| IBIS file stm32h523_533_lqfp100.ibs
[IBIS ver] 4.2
[File name] stm32h523_533_lqfp100.ibs
[File Rev] 0.2
[Date] 07-05-2024
[Source] Data Created at STMicroelectronics
[Notes]  File originated from ELDO simulations.
[Disclaimer]  This information is for modeling purpose only and is
   not guaranteed. The information is subject to change without
   notice.
[Copyright] Copyright 2024 STMicroelectronics Inc.
|   Component stm32h523_533_lqfp100
[Component] stm32h523_533_lqfp100
[Manufacturer] STMicroelectronics
[Package]
| variable   typ   min   max
R_pkg  0  NA  NA
L_pkg  0  NA  NA
C_pkg  0  NA  NA
[Pin]   signal_name   model_name
1  PE2  io8_ft_i3c_spi
2  PE3  io8_ft_i3c_spi
3  PE4  io8_ft_i3c_spi
4  PE5  io8_ft_i3c_spi
5  PE6  io8_ft_i3c_spi
6  VBAT  power
7  PC13  io8_ft_i3c_spi_v33
8  PC14-OSC32_IN  io_ft_tamp
9  PC15-OSC32_OUT  io_ft_tamp
10  VSS  gnd
11  VDD  power
12  PH0-OSC_IN  io8_ft_i3c_spi
13  PH1-OSC_OUT  io8_ft_i3c_spi
14  NRST  ioreset_ft_v33
15  PC0  io8_ft_spi
16  PC1  io8_ft_spi
17  PC2  io8_ft_spi
18  PC3  io8_ft_spi
19  VSSA  nc
20  VREFM  nc
21  VREFP  nc
22  VDDA  nc
23  PA0  io8_ft_spi
24  PA1  io8_ft_spi_tamp
25  PA2  io8_ft_spi
26  PA3  io8_ft_spi
27  VSS  gnd
28  VDD  power
29  PA4  io8_ft_spi
30  PA5  io8_ft_spi
31  PA6  io8_ft_spi
32  PA7  io8_ft_spi
33  PC4  io8_ft_spi
34  PC5  io8_ft_spi
35  PB0  io8_ft_spi
36  PB1  io8_ft_spi
37  PB2  io8_ft_i3c_spi
38  PE7  io8_ft_i3c_spi
39  PE8  io8_ft_i3c_spi
40  PE9  io8_ft_i3c_spi
41  PE10  io8_ft_i3c_spi
42  PE11  io8_ft_i3c_spi
43  PE12  io8_ft_i3c_spi
44  PE13  io8_ft_i3c_spi
45  PE14  io8_ft_i3c_spi
46  PE15  io8_ft_i3c_spi
47  PB10  io8_ft_i3c_spi
48  VCAP  nc
49  VSS  gnd
50  VDD  power
51  PB12  io8_ft_i3c_spi
52  PB13  nc
53  PB14  nc
54  PB15  io8_ft_spi
55  PD8  io8_ft_i3c_spi
56  PD9  io8_ft_i3c_spi
57  PD10  io8_ft_i3c_spi
58  PD11  io8_ft_i3c_spi
59  PD12  io8_ft_i3c_spi
60  PD13  io8_ft_i3c_spi
61  PD14  io8_ft_i3c_spi
62  PD15  io8_ft_i3c_spi
63  PC6  io8_ft_i3c_spi
64  PC7  io8_ft_i3c_spi
65  PC8  io8_ft_i3c_spi
66  PC9  io8_ft_i3c_spi
67  PA8  io8_ft_i3c_spi
68  PA9  io8_ft_i3c_spi
69  PA10  io8_ft_i3c_spi
70  PA11  io8usb_ft_i3c_spi_phy
71  PA12  io8usb_ft_i3c_spi_phy
72  PA13  io8_ft_i3c_spi
73  VDDUSB  power
74  VSS  gnd
75  VDD  power
76  PA14  io8_ft_i3c_spi
77  PA15  io8_ft_i3c_spi
78  PC10  io8_ft_i3c_spi
79  PC11  io8_ft_i3c_spi
80  PC12  io8_ft_i3c_spi
81  PD0  io8_ft_i3c_spi
82  PD1  io8_ft_i3c_spi
83  PD2  io8_ft_i3c_spi
84  PD3  io8_ft_i3c_spi
85  PD4  io8_ft_i3c_spi
86  PD5  io8_ft_i3c_spi
87  PD6  io8_ft_i3c_spi
88  PD7  io8_ft_i3c_spi
89  PB3  io8_ft_i3c_spi
90  PB4  io8_ft_i3c_spi
91  PB5  io8_ft_i3c_spi
92  PB6  io8_ft_i3c_spi
93  PB7  io8_ft_i3c_spi
94  BOOT0  vpphv
95  PB8  io8_ft_i3c_spi
96  PB9  io8_ft_i3c_spi
97  PE0  io8_ft_i3c_spi
98  VCAP  nc
99  VSS  gnd
100  VDD  power
[Package Model]   478-lqfp-14x14-100-240318
[Pin Mapping]   pulldown_ref   pullup_ref   | Comment
1  gndio  vddio
2  gndio  vddio
3  gndio  vddio
4  gndio  vddio
5  gndio  vddio
6  nc  vsw
7  gndio  vddio  | Depending on IO usage
| 7  gndio  vsw  | Depending on IO usage
8  gndio  vddio  | Depending on IO usage
| 8  gndio  vsw  | Depending on IO usage
9  gndio  vddio  | Depending on IO usage
| 9  gndio  vsw  | Depending on IO usage
10  gndio  nc
11  nc  vddio
12  gndio  vddio
13  gndio  vddio
14  gndio  vddio
15  gndio  vddio
16  gndio  vddio
17  gndio  vddio
18  gndio  vddio
19  nc  nc
20  nc  nc
21  nc  nc
22  nc  nc
23  gndio  vddio
24  gndio  vddio
25  gndio  vddio
26  gndio  vddio
27  gndio  nc
28  nc  vddio
29  gndio  vddio
30  gndio  vddio
31  gndio  vddio
32  gndio  vddio
33  gndio  vddio
34  gndio  vddio
35  gndio  vddio
36  gndio  vddio
37  gndio  vddio
38  gndio  vddio
39  gndio  vddio
40  gndio  vddio
41  gndio  vddio
42  gndio  vddio
43  gndio  vddio
44  gndio  vddio
45  gndio  vddio
46  gndio  vddio
47  gndio  vddio
48  nc  nc
49  gndio  nc
50  nc  vddio
51  gndio  vddio
52  nc  nc
53  nc  nc
54  gndio  vddio
55  gndio  vddio
56  gndio  vddio
57  gndio  vddio
58  gndio  vddio
59  gndio  vddio
60  gndio  vddio
61  gndio  vddio
62  gndio  vddio
63  gndio  vddio
64  gndio  vddio
65  gndio  vddio
66  gndio  vddio
67  gndio  vddio
68  gndio  vddio
69  gndio  vddio
70  gndio  vddusb  | Depending on IO usage
| 70  gndio  vddio  | Depending on IO usage
71  gndio  vddusb  | Depending on IO usage
| 71  gndio  vddio  | Depending on IO usage
72  gndio  vddio
73  nc  vddusb
74  gndio  nc
75  nc  vddio
76  gndio  vddio
77  gndio  vddio
78  gndio  vddio
79  gndio  vddio
80  gndio  vddio
81  gndio  vddio
82  gndio  vddio
83  gndio  vddio
84  gndio  vddio
85  gndio  vddio
86  gndio  vddio
87  gndio  vddio
88  gndio  vddio
89  gndio  vddio
90  gndio  vddio
91  gndio  vddio
92  gndio  vddio
93  gndio  vddio
94  gndio  vddio
95  gndio  vddio
96  gndio  vddio
97  gndio  vddio
98  nc  nc
99  gndio  nc
100  nc  vddio
|[Diff Pin]  inv_pin  vdiff  tdelay_typ  tdelay_min  tdelay_max
|71  70  NA  NA  NA  NA
[Model Selector] io8_ft_i3c_spi
io8_ft_spi_ls_1v2 "GPIO SPI - 5V tolerant - low speed - 1.2V range"
io8_ft_spi_ls_1v8 "GPIO SPI - 5V tolerant - low speed - 1.8V range"
io8_ft_spi_ls_3v3 "GPIO SPI - 5V tolerant - low speed - 3.3V range"
io8_ft_spi_ms_1v2 "GPIO SPI - 5V tolerant - med speed - 1.2V range"
io8_ft_spi_ms_1v8 "GPIO SPI - 5V tolerant - med speed - 1.8V range"
io8_ft_spi_ms_3v3 "GPIO SPI - 5V tolerant - med speed - 3.3V range"
io8_ft_spi_fs_1v2 "GPIO SPI - 5V tolerant - fast speed - 1.2V range"
io8_ft_spi_fs_1v8 "GPIO SPI - 5V tolerant - fast speed - 1.8V range"
io8_ft_spi_fs_3v3 "GPIO SPI - 5V tolerant - fast speed - 3.3V range"
io8_ft_spi_hs_1v2 "GPIO SPI - 5V tolerant - high speed - 1.2V range"
io8_ft_spi_hs_1v8 "GPIO SPI - 5V tolerant - high speed - 1.8V range"
io8_ft_spi_hs_3v3 "GPIO SPI - 5V tolerant - high speed - 3.3V range"
io8_ft_hslv_spi_ls_1v2 "GPIO SPI low volt opt - 5V tolerant - low speed - 1.2V range"
io8_ft_hslv_spi_ls_1v8 "GPIO SPI low volt opt - 5V tolerant - low speed - 1.8V range"
io8_ft_hslv_spi_ls_2v5 "GPIO SPI low volt opt - 5V tolerant - low speed - 2.5V range"
io8_ft_hslv_spi_ms_1v2 "GPIO SPI low volt opt - 5V tolerant - med speed - 1.2V range"
io8_ft_hslv_spi_ms_1v8 "GPIO SPI low volt opt - 5V tolerant - med speed - 1.8V range"
io8_ft_hslv_spi_ms_2v5 "GPIO SPI low volt opt - 5V tolerant - med speed - 2.5V range"
io8_ft_hslv_spi_fs_1v2 "GPIO SPI low volt opt - 5V tolerant - fast speed - 1.2V range"
io8_ft_hslv_spi_fs_1v8 "GPIO SPI low volt opt - 5V tolerant - fast speed - 1.8V range"
io8_ft_hslv_spi_fs_2v5 "GPIO SPI low volt opt - 5V tolerant - fast speed - 2.5V range"
io8_ft_hslv_spi_hs_1v2 "GPIO SPI low volt opt - 5V tolerant - high speed - 1.2V range"
io8_ft_hslv_spi_hs_1v8 "GPIO SPI low volt opt - 5V tolerant - high speed - 1.8V range"
io8_ft_hslv_spi_hs_2v5 "GPIO SPI low volt opt - 5V tolerant - high speed - 2.5V range"
io8_ft_i3c_spi_ls_1v2 "GPIO SPI with I3C open-drain - 5V tolerant - low speed - 1.2V range"
io8_ft_i3c_spi_ls_1v8 "GPIO SPI with I3C open-drain - 5V tolerant - low speed - 1.8V range"
io8_ft_i3c_spi_ls_3v3 "GPIO SPI with I3C open-drain - 5V tolerant - low speed - 3.3V range"
io8_ft_i3c_spi_ms_1v2 "GPIO SPI with I3C open-drain - 5V tolerant - med speed - 1.2V range"
io8_ft_i3c_spi_ms_1v8 "GPIO SPI with I3C open-drain - 5V tolerant - med speed - 1.8V range"
io8_ft_i3c_spi_ms_3v3 "GPIO SPI with I3C open-drain - 5V tolerant - med speed - 3.3V range"
io8_ft_i3c_spi_fs_1v2 "GPIO SPI with I3C open-drain - 5V tolerant - fast speed - 1.2V range"
io8_ft_i3c_spi_fs_1v8 "GPIO SPI with I3C open-drain - 5V tolerant - fast speed - 1.8V range"
io8_ft_i3c_spi_fs_3v3 "GPIO SPI with I3C open-drain - 5V tolerant - fast speed - 3.3V range"
io8_ft_i3c_spi_hs_1v2 "GPIO SPI with I3C open-drain - 5V tolerant - high speed - 1.2V range"
io8_ft_i3c_spi_hs_1v8 "GPIO SPI with I3C open-drain - 5V tolerant - high speed - 1.8V range"
io8_ft_i3c_spi_hs_3v3 "GPIO SPI with I3C open-drain - 5V tolerant - high speed - 3.3V range"
io8_ft_hslv_i3c_spi_ls_1v2 "GPIO SPI low volt opt with I3C open-drain - 5V tolerant - low speed - 1.2V range"
io8_ft_hslv_i3c_spi_ls_1v8 "GPIO SPI low volt opt with I3C open-drain - 5V tolerant - low speed - 1.8V range"
io8_ft_hslv_i3c_spi_ls_2v5 "GPIO SPI low volt opt with I3C open-drain - 5V tolerant - low speed - 2.5V range"
io8_ft_hslv_i3c_spi_ms_1v2 "GPIO SPI low volt opt with I3C open-drain - 5V tolerant - med speed - 1.2V range"
io8_ft_hslv_i3c_spi_ms_1v8 "GPIO SPI low volt opt with I3C open-drain - 5V tolerant - med speed - 1.8V range"
io8_ft_hslv_i3c_spi_ms_2v5 "GPIO SPI low volt opt with I3C open-drain - 5V tolerant - med speed - 2.5V range"
io8_ft_hslv_i3c_spi_fs_1v2 "GPIO SPI low volt opt with I3C open-drain - 5V tolerant - fast speed - 1.2V range"
io8_ft_hslv_i3c_spi_fs_1v8 "GPIO SPI low volt opt with I3C open-drain - 5V tolerant - fast speed - 1.8V range"
io8_ft_hslv_i3c_spi_fs_2v5 "GPIO SPI low volt opt with I3C open-drain - 5V tolerant - fast speed - 2.5V range"
io8_ft_hslv_i3c_spi_hs_1v2 "GPIO SPI low volt opt with I3C open-drain - 5V tolerant - high speed - 1.2V range"
io8_ft_hslv_i3c_spi_hs_1v8 "GPIO SPI low volt opt with I3C open-drain - 5V tolerant - high speed - 1.8V range"
io8_ft_hslv_i3c_spi_hs_2v5 "GPIO SPI low volt opt with I3C open-drain - 5V tolerant - high speed - 2.5V range"
io8_ft_i3c_fmp_spi_3v3 "GPIO SPI with I3C fm+ open-drain - 5V tolerant - 3.3V range"
io8_ft_i3c_fmp_spi_1v8 "GPIO SPI with I3C fm+ open-drain - 5V tolerant - 1.8V range"
io8_ft_i3c_fmp_spi_1v2 "GPIO SPI with I3C fm+ open-drain - 5V tolerant - 1.2V range"
[Model Selector] io8_ft_i3c_spi_v33
io8_ft_spi_v33_ls_1v2 ""GPIO SPI V33 - 5V tolerant - low speed - 1.2V range"
io8_ft_spi_v33_ls_1v8 ""GPIO SPI V33 - 5V tolerant - low speed - 1.8V range"
io8_ft_spi_v33_ls_3v3 ""GPIO SPI V33 - 5V tolerant - low speed - 3.3V range"
io8_ft_spi_v33_ms_1v2 ""GPIO SPI V33 - 5V tolerant - med speed - 1.2V range"
io8_ft_spi_v33_ms_1v8 ""GPIO SPI V33 - 5V tolerant - med speed - 1.8V range"
io8_ft_spi_v33_ms_3v3 ""GPIO SPI V33 - 5V tolerant - med speed - 3.3V range"
io8_ft_spi_v33_fs_1v2 ""GPIO SPI V33 - 5V tolerant - fast speed - 1.2V range
io8_ft_spi_v33_fs_1v8 ""GPIO SPI V33 - 5V tolerant - fast speed - 1.8V range
io8_ft_spi_v33_fs_3v3 ""GPIO SPI V33 - 5V tolerant - fast speed - 3.3V range
io8_ft_spi_v33_hs_1v2 ""GPIO SPI V33 - 5V tolerant - high speed - 1.2V range
io8_ft_spi_v33_hs_1v8 ""GPIO SPI V33 - 5V tolerant - high speed - 1.8V range
io8_ft_spi_v33_hs_3v3 ""GPIO SPI V33 - 5V tolerant - high speed - 3.3V range
io8_ft_hslv_spi_v33_ls_1v2 "GPIO SPI V33 low volt opt - 5V tolerant - low speed - 1.2V range""
io8_ft_hslv_spi_v33_ls_1v8 "GPIO SPI V33 low volt opt - 5V tolerant - low speed - 1.8V range""
io8_ft_hslv_spi_v33_ls_2v5 "GPIO SPI V33 low volt opt - 5V tolerant - low speed - 2.5V range""
io8_ft_hslv_spi_v33_ms_1v2 "GPIO SPI V33 low volt opt - 5V tolerant - med speed - 1.2V range""
io8_ft_hslv_spi_v33_ms_1v8 "GPIO SPI V33 low volt opt - 5V tolerant - med speed - 1.8V range""
io8_ft_hslv_spi_v33_ms_2v5 "GPIO SPI V33 low volt opt - 5V tolerant - med speed - 2.5V range""
io8_ft_hslv_spi_v33_fs_1v2 "GPIO SPI V33 low volt opt - 5V tolerant - fast speed - 1.2V range"
io8_ft_hslv_spi_v33_fs_1v8 "GPIO SPI V33 low volt opt - 5V tolerant - fast speed - 1.8V range"
io8_ft_hslv_spi_v33_fs_2v5 "GPIO SPI V33 low volt opt - 5V tolerant - fast speed - 2.5V range"
io8_ft_hslv_spi_v33_hs_1v2 "GPIO SPI V33 low volt opt - 5V tolerant - high speed - 1.2V range"
io8_ft_hslv_spi_v33_hs_1v8 "GPIO SPI V33 low volt opt - 5V tolerant - high speed - 1.8V range"
io8_ft_hslv_spi_v33_hs_2v5 "GPIO SPI V33 low volt opt - 5V tolerant - high speed - 2.5V range"
io8_ft_i3c_spi_v33_ls_1v2 "GPIO SPI V33 with I3C open-drain - 5V tolerant - low speed - 1.2V range"
io8_ft_i3c_spi_v33_ls_1v8 "GPIO SPI V33 with I3C open-drain - 5V tolerant - low speed - 1.8V range"
io8_ft_i3c_spi_v33_ls_3v3 "GPIO SPI V33 with I3C open-drain - 5V tolerant - low speed - 3.3V range"
io8_ft_i3c_spi_v33_ms_1v2 "GPIO SPI V33 with I3C open-drain - 5V tolerant - med speed - 1.2V range"
io8_ft_i3c_spi_v33_ms_1v8 "GPIO SPI V33 with I3C open-drain - 5V tolerant - med speed - 1.8V range"
io8_ft_i3c_spi_v33_ms_3v3 "GPIO SPI V33 with I3C open-drain - 5V tolerant - med speed - 3.3V range"
io8_ft_i3c_spi_v33_fs_1v2 "GPIO SPI V33 with I3C open-drain - 5V tolerant - fast speed - 1.2V range"
io8_ft_i3c_spi_v33_fs_1v8 "GPIO SPI V33 with I3C open-drain - 5V tolerant - fast speed - 1.8V range"
io8_ft_i3c_spi_v33_fs_3v3 "GPIO SPI V33 with I3C open-drain - 5V tolerant - fast speed - 3.3V range"
io8_ft_i3c_spi_v33_hs_1v2 "GPIO SPI V33 with I3C open-drain - 5V tolerant - high speed - 1.2V range"
io8_ft_i3c_spi_v33_hs_1v8 "GPIO SPI V33 with I3C open-drain - 5V tolerant - high speed - 1.8V range"
io8_ft_i3c_spi_v33_hs_3v3 "GPIO SPI V33 with I3C open-drain - 5V tolerant - high speed - 3.3V range"
io8_ft_hslv_i3c_spi_v33_ls_1v2 "GPIO SPI V33 low volt opt with I3C open-drain - 5V tolerant - low speed - 1.2V range"
io8_ft_hslv_i3c_spi_v33_ls_1v8 "GPIO SPI V33 low volt opt with I3C open-drain - 5V tolerant - low speed - 1.8V range"
io8_ft_hslv_i3c_spi_v33_ls_2v5 "GPIO SPI V33 low volt opt with I3C open-drain - 5V tolerant - low speed - 2.5V range"
io8_ft_hslv_i3c_spi_v33_ms_1v2 "GPIO SPI V33 low volt opt with I3C open-drain - 5V tolerant - med speed - 1.2V range"
io8_ft_hslv_i3c_spi_v33_ms_1v8 "GPIO SPI V33 low volt opt with I3C open-drain - 5V tolerant - med speed - 1.8V range"
io8_ft_hslv_i3c_spi_v33_ms_2v5 "GPIO SPI V33 low volt opt with I3C open-drain - 5V tolerant - med speed - 2.5V range"
io8_ft_hslv_i3c_spi_v33_fs_1v2 "GPIO SPI V33 low volt opt with I3C open-drain - 5V tolerant - fast speed - 1.2V range"
io8_ft_hslv_i3c_spi_v33_fs_1v8 "GPIO SPI V33 low volt opt with I3C open-drain - 5V tolerant - fast speed - 1.8V range"
io8_ft_hslv_i3c_spi_v33_fs_2v5 "GPIO SPI V33 low volt opt with I3C open-drain - 5V tolerant - fast speed - 2.5V range"
io8_ft_hslv_i3c_spi_v33_hs_1v2 "GPIO SPI V33 low volt opt with I3C open-drain - 5V tolerant - high speed - 1.2V range"
io8_ft_hslv_i3c_spi_v33_hs_1v8 "GPIO SPI V33 low volt opt with I3C open-drain - 5V tolerant - high speed - 1.8V range"
io8_ft_hslv_i3c_spi_v33_hs_2v5 "GPIO SPI V33 low volt opt with I3C open-drain - 5V tolerant - high speed - 2.5V range"
io8_ft_i3c_fmp_spi_v33_3v3 "GPIO SPI V33 with I3C fm+ open-drain - 5V tolerant - 3.3V range"
io8_ft_i3c_fmp_spi_v33_1v8 "GPIO SPI V33 with I3C fm+ open-drain - 5V tolerant - 1.8V range"
io8_ft_i3c_fmp_spi_v33_1v2 "GPIO SPI V33 with I3C fm+ open-drain - 5V tolerant - 1.2V range"
[Model Selector] io8_ft_spi
io8_ft_spi_ls_1v2 "GPIO SPI - 5V tolerant - low speed - 1.2V range"
io8_ft_spi_ls_1v8 "GPIO SPI - 5V tolerant - low speed - 1.8V range"
io8_ft_spi_ls_3v3 "GPIO SPI - 5V tolerant - low speed - 3.3V range"
io8_ft_spi_ms_1v2 "GPIO SPI- 5V tolerant - med speed - 1.2V range"
io8_ft_spi_ms_1v8 "GPIO SPI- 5V tolerant - med speed - 1.8V range"
io8_ft_spi_ms_3v3 "GPIO SPI- 5V tolerant - med speed - 3.3V range"
io8_ft_spi_fs_1v2 "GPIO SPI- 5V tolerant - fast speed - 1.2V range"
io8_ft_spi_fs_1v8 "GPIO SPI- 5V tolerant - fast speed - 1.8V range"
io8_ft_spi_fs_3v3 "GPIO SPI- 5V tolerant - fast speed - 3.3V range"
io8_ft_spi_hs_1v2 "GPIO SPI- 5V tolerant - high speed - 1.2V range"
io8_ft_spi_hs_1v8 "GPIO SPI- 5V tolerant - high speed - 1.8V range"
io8_ft_spi_hs_3v3 "GPIO SPI- 5V tolerant - high speed - 3.3V range"
io8_ft_hslv_spi_ls_1v2 "GPIO SPI low volt opt - 5V tolerant - low speed - 1.2V range"
io8_ft_hslv_spi_ls_1v8 "GPIO SPI low volt opt - 5V tolerant - low speed - 1.8V range"
io8_ft_hslv_spi_ls_2v5 "GPIO SPI low volt opt - 5V tolerant - low speed - 2.5V range"
io8_ft_hslv_spi_ms_1v2 "GPIO SPI low volt opt - 5V tolerant - med speed - 1.2V range"
io8_ft_hslv_spi_ms_1v8 "GPIO SPI low volt opt - 5V tolerant - med speed - 1.8V range"
io8_ft_hslv_spi_ms_2v5 "GPIO SPI low volt opt - 5V tolerant - med speed - 2.5V range"
io8_ft_hslv_spi_fs_1v2 "GPIO SPI low volt opt - 5V tolerant - fast speed - 1.2V range"
io8_ft_hslv_spi_fs_1v8 "GPIO SPI low volt opt - 5V tolerant - fast speed - 1.8V range"
io8_ft_hslv_spi_fs_2v5 "GPIO SPI low volt opt - 5V tolerant - fast speed - 2.5V range"
io8_ft_hslv_spi_hs_1v2 "GPIO SPI low volt opt - 5V tolerant - high speed - 1.2V range"
io8_ft_hslv_spi_hs_1v8 "GPIO SPI low volt opt - 5V tolerant - high speed - 1.8V range"
io8_ft_hslv_spi_hs_2v5 "GPIO SPI low volt opt - 5V tolerant - high speed - 2.5V range"
[Model Selector] io8_ft_spi_tamp
io8_ft_spi_ls_1v2 "GPIO SPI - 5V tolerant - low speed - 1.2V range"
io8_ft_spi_ls_1v8 "GPIO SPI - 5V tolerant - low speed - 1.8V range"
io8_ft_spi_ls_3v3 "GPIO SPI- 5V tolerant - low speed - 3.3V range"
io8_ft_spi_ms_1v2 "GPIO SPI - 5V tolerant - med speed - 1.2V range"
io8_ft_spi_ms_1v8 "GPIO SPI - 5V tolerant - med speed - 1.8V range"
io8_ft_spi_ms_3v3 "GPIO SPI - 5V tolerant - med speed - 3.3V range"
io8_ft_spi_fs_1v2 "GPIO SPI - 5V tolerant - fast speed - 1.2V range"
io8_ft_spi_fs_1v8 "GPIO SPI - 5V tolerant - fast speed - 1.8V range"
io8_ft_spi_fs_3v3 "GPIO SPI - 5V tolerant - fast speed - 3.3V range"
io8_ft_spi_hs_1v2 "GPIO SPI - 5V tolerant - high speed - 1.2V range"
io8_ft_spi_hs_1v8 "GPIO SPI - 5V tolerant - high speed - 1.8V range"
io8_ft_spi_hs_3v3 "GPIO SPI - 5V tolerant - high speed - 3.3V range"
io8_ft_hslv_spi_ls_1v2 "GPIO SPI low volt opt - 5V tolerant - low speed - 1.2V range"
io8_ft_hslv_spi_ls_1v8 "GPIO SPI low volt opt - 5V tolerant - low speed - 1.8V range"
io8_ft_hslv_spi_ls_2v5 "GPIO SPI low volt opt - 5V tolerant - low speed - 2.5V range"
io8_ft_hslv_spi_ms_1v2 "GPIO SPI low volt opt - 5V tolerant - med speed - 1.2V range"
io8_ft_hslv_spi_ms_1v8 "GPIO SPI low volt opt - 5V tolerant - med speed - 1.8V range"
io8_ft_hslv_spi_ms_2v5 "GPIO SPI low volt opt - 5V tolerant - med speed - 2.5V range"
io8_ft_hslv_spi_fs_1v2 "GPIO SPI low volt opt - 5V tolerant - fast speed - 1.2V range"
io8_ft_hslv_spi_fs_1v8 "GPIO SPI low volt opt - 5V tolerant - fast speed - 1.8V range"
io8_ft_hslv_spi_fs_2v5 "GPIO SPI low volt opt - 5V tolerant - fast speed - 2.5V range"
io8_ft_hslv_spi_hs_1v2 "GPIO SPI low volt opt - 5V tolerant - high speed - 1.2V range"
io8_ft_hslv_spi_hs_1v8 "GPIO SPI low volt opt - 5V tolerant - high speed - 1.8V range"
io8_ft_hslv_spi_hs_2v5 "GPIO SPI low volt opt - 5V tolerant - high speed - 2.5V range
io8_ft_tamp_v33_1v2 "IO tamper - 5V tolerant - 1.2V range"
io8_ft_tamp_v33_1v8 "IO tamper - 5V tolerant - 1.8V range"
io8_ft_tamp_v33_3v3 "IO tamper - 5V tolerant - 3.3V range"
[Model Selector] io8usb_ft_i3c_spi_phy
io8_ft_spi_ls_1v2 "GPIO SPI - 5V tolerant - low speed - 1.2V range"
io8_ft_spi_ls_1v8 "GPIO SPI - 5V tolerant - low speed - 1.8V range"
io8_ft_spi_ls_3v3 "GPIO SPI - 5V tolerant - low speed - 3.3V range"
io8_ft_spi_ms_1v2 "GPIO SPI - 5V tolerant - med speed - 1.2V range"
io8_ft_spi_ms_1v8 "GPIO SPI - 5V tolerant - med speed - 1.8V range"
io8_ft_spi_ms_3v3 "GPIO SPI - 5V tolerant - med speed - 3.3V range"
io8_ft_spi_fs_1v2 "GPIO SPI - 5V tolerant - fast speed - 1.2V range"
io8_ft_spi_fs_1v8 "GPIO SPI - 5V tolerant - fast speed - 1.8V range"
io8_ft_spi_fs_3v3 "GPIO SPI - 5V tolerant - fast speed - 3.3V range"
io8_ft_spi_hs_1v2 "GPIO SPI - 5V tolerant - high speed - 1.2V range"
io8_ft_spi_hs_1v8 "GPIO SPI - 5V tolerant - high speed - 1.8V range"
io8_ft_spi_hs_3v3 "GPIO SPI - 5V tolerant - high speed - 3.3V range"
io8_ft_hslv_spi_ls_1v2 "GPIO SPI low volt opt - 5V tolerant - low speed - 1.2V range"
io8_ft_hslv_spi_ls_1v8 "GPIO SPI low volt opt - 5V tolerant - low speed - 1.8V range"
io8_ft_hslv_spi_ls_2v5 "GPIO SPI low volt opt - 5V tolerant - low speed - 2.5V range"
io8_ft_hslv_spi_ms_1v2 "GPIO SPI low volt opt - 5V tolerant - med speed - 1.2V range"
io8_ft_hslv_spi_ms_1v8 "GPIO SPI low volt opt - 5V tolerant - med speed - 1.8V range"
io8_ft_hslv_spi_ms_2v5 "GPIO SPI low volt opt - 5V tolerant - med speed - 2.5V range"
io8_ft_hslv_spi_fs_1v2 "GPIO SPI low volt opt - 5V tolerant - fast speed - 1.2V range"
io8_ft_hslv_spi_fs_1v8 "GPIO SPI low volt opt - 5V tolerant - fast speed - 1.8V range"
io8_ft_hslv_spi_fs_2v5 "GPIO SPI low volt opt - 5V tolerant - fast speed - 2.5V range"
io8_ft_hslv_spi_hs_1v2 "GPIO SPI low volt opt - 5V tolerant - high speed - 1.2V range"
io8_ft_hslv_spi_hs_1v8 "GPIO SPI low volt opt - 5V tolerant - high speed - 1.8V range"
io8_ft_hslv_spi_hs_2v5 "GPIO SPI low volt opt - 5V tolerant - high speed - 2.5V range"
io8_ft_i3c_spi_ls_1v2 "GPIO SPI  with I3C open-drain - 5V tolerant - low speed - 1.2V range"
io8_ft_i3c_spi_ls_1v8 "GPIO SPI  with I3C open-drain - 5V tolerant - low speed - 1.8V range"
io8_ft_i3c_spi_ls_3v3 "GPIO SPI  with I3C open-drain - 5V tolerant - low speed - 3.3V range"
io8_ft_i3c_spi_ms_1v2 "GPIO SPI  with I3C open-drain - 5V tolerant - med speed - 1.2V range"
io8_ft_i3c_spi_ms_1v8 "GPIO SPI  with I3C open-drain - 5V tolerant - med speed - 1.8V range"
io8_ft_i3c_spi_ms_3v3 "GPIO SPI  with I3C open-drain - 5V tolerant - med speed - 3.3V range"
io8_ft_i3c_spi_fs_1v2 "GPIO SPI  with I3C open-drain - 5V tolerant - fast speed - 1.2V range"
io8_ft_i3c_spi_fs_1v8 "GPIO SPI  with I3C open-drain - 5V tolerant - fast speed - 1.8V range"
io8_ft_i3c_spi_fs_3v3 "GPIO SPI  with I3C open-drain - 5V tolerant - fast speed - 3.3V range"
io8_ft_i3c_spi_hs_1v2 "GPIO SPI  with I3C open-drain - 5V tolerant - high speed - 1.2V range"
io8_ft_i3c_spi_hs_1v8 "GPIO SPI  with I3C open-drain - 5V tolerant - high speed - 1.8V range"
io8_ft_i3c_spi_hs_3v3 "GPIO SPI  with I3C open-drain - 5V tolerant - high speed - 3.3V range"
io8_ft_hslv_i3c_spi_ls_1v2 "GPIO SPI  low volt opt with I3C open-drain - 5V tolerant - low speed - 1.2V range"
io8_ft_hslv_i3c_spi_ls_1v8 "GPIO SPI  low volt opt with I3C open-drain - 5V tolerant - low speed - 1.8V range"
io8_ft_hslv_i3c_spi_ls_2v5 "GPIO SPI  low volt opt with I3C open-drain - 5V tolerant - low speed - 2.5V range"
io8_ft_hslv_i3c_spi_ms_1v2 "GPIO SPI  low volt opt with I3C open-drain - 5V tolerant - med speed - 1.2V range"
io8_ft_hslv_i3c_spi_ms_1v8 "GPIO SPI  low volt opt with I3C open-drain - 5V tolerant - med speed - 1.8V range"
io8_ft_hslv_i3c_spi_ms_2v5 "GPIO SPI  low volt opt with I3C open-drain - 5V tolerant - med speed - 2.5V range"
io8_ft_hslv_i3c_spi_fs_1v2 "GPIO SPI  low volt opt with I3C open-drain - 5V tolerant - fast speed - 1.2V range"
io8_ft_hslv_i3c_spi_fs_1v8 "GPIO SPI  low volt opt with I3C open-drain - 5V tolerant - fast speed - 1.8V range"
io8_ft_hslv_i3c_spi_fs_2v5 "GPIO SPI  low volt opt with I3C open-drain - 5V tolerant - fast speed - 2.5V range"
io8_ft_hslv_i3c_spi_hs_1v2 "GPIO SPI  low volt opt with I3C open-drain - 5V tolerant - high speed - 1.2V range"
io8_ft_hslv_i3c_spi_hs_1v8 "GPIO SPI  low volt opt with I3C open-drain - 5V tolerant - high speed - 1.8V range"
io8_ft_hslv_i3c_spi_hs_2v5 "GPIO SPI  low volt opt with I3C open-drain - 5V tolerant - high speed - 2.5V range"
io8_ft_i3c_fmp_spi_3v3 "GPIO SPI  with I3C fm+ open-drain - 5V tolerant - 3.3V range"
io8_ft_i3c_fmp_spi_1v8 "GPIO SPI  with I3C fm+ open-drain - 5V tolerant - 1.8V range"
io8_ft_i3c_fmp_spi_1v2 "GPIO SPI  with I3C fm+ open-drain - 5V tolerant - 1.2V range"
io8usb_ft_phy_ls_2v5 "USB PHY - 5V tolerant - low speed - 2.5V range"
io8usb_ft_phy_ls_3v3 "USB PHY - 5V tolerant - low speed - 3.3V range
io8usb_ft_phy_fs_2v5 "USB PHY - 5V tolerant - fast speed - 2.5V range"
io8usb_ft_phy_fs_3v3 "USB PHY - 5V tolerant - fast speed - 3.3V range"
[Model Selector] io_ft_tamp
io_ft_tamp_3v3 "IO tamper - 5V tolerant - 3.3V range"
io_ft_tamp_1v8 "IO tamper - 5V tolerant - 1.8V range"
io_ft_tamp_1v2 "IO tamper - 5V tolerant - 1.2V range"
[Model Selector] ioreset_ft_v33
ioreset_ft_v33_1v2 "Reset PAD. 5V tolerant. 1.2V range"
ioreset_ft_v33_1v8 "Reset PAD. 5V tolerant. 1.8V range"
ioreset_ft_v33_3v3 "Reset PAD. 5V tolerant. 3.3V range"
[Model Selector] vpphv
vpphv_1v2 "Flash Test cell v33 = 1.2 V range"
vpphv_1v8 "Flash Test cell v33 = 1.8 V range"
vpphv_3v3 "Flash Test cell v33 = 3.3 V range"
[Define Package Model]  478-lqfp-14x14-100-240318
[Manufacturer]  Unknown
[OEM]  Unknown
[Description]  None
[Number Of Pins]  96
[Pin Numbers]
| Pin Num   Terminal Name
14 | NRST
23 | PA0
24 | PA1
25 | PA2
26 | PA3
29 | PA4
30 | PA5
31 | PA6
32 | PA7
67 | PA8
68 | PA9
69 | PA10
70 | PA11
71 | PA12
72 | PA13
76 | PA14
77 | PA15
35 | PB0
36 | PB1
37 | PB2
89 | PB3
90 | PB4
91 | PB5
92 | PB6
93 | PB7
95 | PB8
96 | PB9
47 | PB10
51 | PB12
52 | PB13
53 | PB14
54 | PB15
15 | PC0
16 | PC1
17 | PC2
18 | PC3
33 | PC4
34 | PC5
63 | PC6
64 | PC7
65 | PC8
66 | PC9
78 | PC10
79 | PC11
80 | PC12
7 | PC13
8 | PC14-OSC32_IN
9 | PC15-OSC32_OUT
81 | PD0
82 | PD1
83 | PD2
84 | PD3
85 | PD4
86 | PD5
87 | PD6
88 | PD7
55 | PD8
56 | PD9
57 | PD10
58 | PD11
59 | PD12
60 | PD13
61 | PD14
62 | PD15
97 | PE0
1 | PE2
2 | PE3
3 | PE4
4 | PE5
5 | PE6
38 | PE7
39 | PE8
40 | PE9
41 | PE10
42 | PE11
43 | PE12
44 | PE13
45 | PE14
46 | PE15
12 | PH0-OSC_IN
13 | PH1-OSC_OUT
6 | VBAT
48 | VCAP
98 | VCAP
50 | VDD
75 | VDD
11 | VDD
28 | VDD
100 | VDD
73 | VDDUSB
22 | VDDA
94 | BOOT0
20 | VREFM
21 | VREFP
10 | VSS
19 | VSSA
|[Merged Pins]  10
|27  |  VSS
|49  |  VSS
|74  |  VSS
|99  |  VSS
[Model Data]
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[End Model Data]
[End Package Model]
|End [Component]
| Models and submodels in the file (118): io8_ft_hslv_i3c_spi_fs_1v2 (I/O_open_drain), io8_ft_hslv_i3c_spi_fs_1v8 (I/O_open_drain), io8_ft_hslv_i3c_spi_fs_2v5 (I/O_open_drain), io8_ft_hslv_i3c_spi_hs_1v2 (I/O_open_drain), io8_ft_hslv_i3c_spi_hs_1v8 (I/O_open_drain), io8_ft_hslv_i3c_spi_hs_2v5 (I/O_open_drain), io8_ft_hslv_i3c_spi_ls_1v2 (I/O_open_drain), io8_ft_hslv_i3c_spi_ls_1v8 (I/O_open_drain), io8_ft_hslv_i3c_spi_ls_2v5 (I/O_open_drain), io8_ft_hslv_i3c_spi_ms_1v2 (I/O_open_drain), io8_ft_hslv_i3c_spi_ms_1v8 (I/O_open_drain), io8_ft_hslv_i3c_spi_ms_2v5 (I/O_open_drain), io8_ft_hslv_i3c_spi_v33_fs_1v2 (I/O_open_drain), io8_ft_hslv_i3c_spi_v33_fs_1v8 (I/O_open_drain), io8_ft_hslv_i3c_spi_v33_fs_2v5 (I/O_open_drain), io8_ft_hslv_i3c_spi_v33_hs_1v2 (I/O_open_drain), io8_ft_hslv_i3c_spi_v33_hs_1v8 (I/O_open_drain), io8_ft_hslv_i3c_spi_v33_hs_2v5 (I/O_open_drain), io8_ft_hslv_i3c_spi_v33_ls_1v2 (I/O_open_drain), io8_ft_hslv_i3c_spi_v33_ls_1v8 (I/O_open_drain), io8_ft_hslv_i3c_spi_v33_ls_2v5 (I/O_open_drain), io8_ft_hslv_i3c_spi_v33_ms_1v2 (I/O_open_drain), io8_ft_hslv_i3c_spi_v33_ms_1v8 (I/O_open_drain), io8_ft_hslv_i3c_spi_v33_ms_2v5 (I/O_open_drain), io8_ft_hslv_spi_fs_1v2 (I/O), io8_ft_hslv_spi_fs_1v8 (I/O), io8_ft_hslv_spi_fs_2v5 (I/O), io8_ft_hslv_spi_hs_1v2 (I/O), io8_ft_hslv_spi_hs_1v8 (I/O), io8_ft_hslv_spi_hs_2v5 (I/O), io8_ft_hslv_spi_ls_1v2 (I/O), io8_ft_hslv_spi_ls_1v8 (I/O), io8_ft_hslv_spi_ls_2v5 (I/O), io8_ft_hslv_spi_ms_1v2 (I/O), io8_ft_hslv_spi_ms_1v8 (I/O), io8_ft_hslv_spi_ms_2v5 (I/O), io8_ft_hslv_spi_v33_fs_1v2 (I/O), io8_ft_hslv_spi_v33_fs_1v8 (I/O), io8_ft_hslv_spi_v33_fs_2v5 (I/O), io8_ft_hslv_spi_v33_hs_1v2 (I/O), io8_ft_hslv_spi_v33_hs_1v8 (I/O), io8_ft_hslv_spi_v33_hs_2v5 (I/O), io8_ft_hslv_spi_v33_ls_1v2 (I/O), io8_ft_hslv_spi_v33_ls_1v8 (I/O), io8_ft_hslv_spi_v33_ls_2v5 (I/O), io8_ft_hslv_spi_v33_ms_1v2 (I/O), io8_ft_hslv_spi_v33_ms_1v8 (I/O), io8_ft_hslv_spi_v33_ms_2v5 (I/O), io8_ft_i3c_fmp_spi_1v2 (I/O_open_drain), io8_ft_i3c_fmp_spi_1v8 (I/O_open_drain), io8_ft_i3c_fmp_spi_3v3 (I/O_open_drain), io8_ft_i3c_fmp_spi_v33_1v2 (I/O_open_drain), io8_ft_i3c_fmp_spi_v33_1v8 (I/O_open_drain), io8_ft_i3c_fmp_spi_v33_3v3 (I/O_open_drain), io8_ft_i3c_spi_fs_1v2 (I/O_open_drain), io8_ft_i3c_spi_fs_1v8 (I/O_open_drain), io8_ft_i3c_spi_fs_3v3 (I/O_open_drain), io8_ft_i3c_spi_hs_1v2 (I/O_open_drain), io8_ft_i3c_spi_hs_1v8 (I/O_open_drain), io8_ft_i3c_spi_hs_3v3 (I/O_open_drain), io8_ft_i3c_spi_ls_1v2 (I/O_open_drain), io8_ft_i3c_spi_ls_1v8 (I/O_open_drain), io8_ft_i3c_spi_ls_3v3 (I/O_open_drain), io8_ft_i3c_spi_ms_1v2 (I/O_open_drain), io8_ft_i3c_spi_ms_1v8 (I/O_open_drain), io8_ft_i3c_spi_ms_3v3 (I/O_open_drain), io8_ft_i3c_spi_v33_fs_1v2 (I/O_open_drain), io8_ft_i3c_spi_v33_fs_1v8 (I/O_open_drain), io8_ft_i3c_spi_v33_fs_3v3 (I/O_open_drain), io8_ft_i3c_spi_v33_hs_1v2 (I/O_open_drain), io8_ft_i3c_spi_v33_hs_1v8 (I/O_open_drain), io8_ft_i3c_spi_v33_hs_3v3 (I/O_open_drain), io8_ft_i3c_spi_v33_ls_1v2 (I/O_open_drain), io8_ft_i3c_spi_v33_ls_1v8 (I/O_open_drain), io8_ft_i3c_spi_v33_ls_3v3 (I/O_open_drain), io8_ft_i3c_spi_v33_ms_1v2 (I/O_open_drain), io8_ft_i3c_spi_v33_ms_1v8 (I/O_open_drain), io8_ft_i3c_spi_v33_ms_3v3 (I/O_open_drain), io8_ft_spi_fs_1v2 (I/O), io8_ft_spi_fs_1v8 (I/O)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
